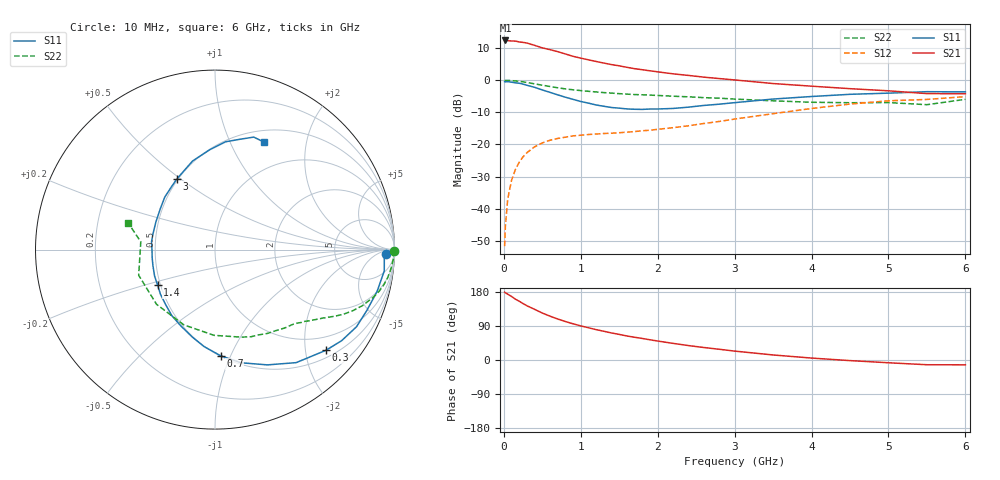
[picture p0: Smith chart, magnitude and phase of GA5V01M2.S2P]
! Infineon Technologies  Discrete & RF Semiconductors
! BF775
! Si NPN RF Bipolar Junction Transistor in SOT23
! VCE = 5 V  IC = 1.2 mA
! Common Emitter S-Parameters:  May  1996
# GHz  S  MA  R  50
!  f  S11  S21  S12  S22
! GHz  MAG  ANG  MAG  ANG  MAG  ANG  MAG  ANG
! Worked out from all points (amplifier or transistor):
!   36 points, 10 MHz to 6 GHz, reference 50 ohm
!   highest |S21| = 12.4 dB at 20 MHz (marker M1)
!   |S21| within 3 dB of that: start of sweep to 622.2 MHz
!   unconditionally stable (mu >= 1): 1.385 GHz to 3.704 GHz; 5.262 GHz to end of sweep
!   at 250 MHz: K = 0.21, MSG = 17.8 dB, |S12| = -23.8 dB
!   at 1.4 GHz: K = 1.01, MAG = 10.1 dB, |S12| = -16.5 dB
!   at 6 GHz: K = 1.00, MAG = 0.3 dB, |S12| = -5.1 dB
!   S11 on the Smith chart (normalised r, x): 10 MHz: 32, -17; 300 MHz: 0.66, -2.44; 700 MHz: 0.50, -0.92; 1.4 GHz: 0.48, -0.22; 3 GHz: 0.49, +0.48; 6 GHz: 0.64, +1.35
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0.01  0.9516 -1.5  4.094 179.0  0.0026 88.5  0.9999 -0.5
0.02  0.9444 -2.7  4.165 177.4  0.0053 92.0  0.9907 -1.2
0.05  0.9505 -7.2  4.133 173.8  0.014 85.1  0.9946 -3.1
0.1  0.9326 -14.5  4.084 167.7  0.0276 81.3  0.9867 -6.0
0.15  0.9113 -21.9  4.071 160.6  0.0406 76.4  0.975 -9.2
0.3  0.8349 -42.2  3.798 143.1  0.0744 65.2  0.9208 -16.8
0.4  0.7754 -54.3  3.493 133.7  0.0917 58.7  0.8779 -20.9
0.5  0.7058 -65.5  3.193 123.9  0.1055 53.5  0.8375 -24.1
0.6  0.6472 -77.0  2.996 115.6  0.1162 49.2  0.7986 -26.9
0.7  0.5921 -87.0  2.788 108.2  0.124 45.9  0.7631 -29.1
0.8  0.5438 -96.4  2.565 101.5  0.1297 43.1  0.7325 -31.0
0.9  0.5035 -104.5  2.358 95.5  0.1359 41.1  0.7094 -32.6
1.1  0.4398 -123.1  2.079 85.1  0.1427 38.7  0.6726 -35.7
1.4  0.3757 -148.5  1.752 71.3  0.1495 37.8  0.6301 -40.1
1.7  0.353 -172.6  1.514 60.0  0.1586 39.6  0.598 -44.5
2.2  0.3635 155.0  1.258 43.9  0.1823 43.5  0.5636 -53.4
3  0.4474 118.4  1.011 23.5  0.2482 46.3  0.5089 -73.4
3.5  0.5093 104.2  0.888 13.3  0.3014 44.0  0.4778 -90.6
4.5  0.6035 84.4  0.739 -1.6  0.4251 32.9  0.4461 -136.9
5  0.6292 77.5  0.684 -7.3  0.4783 24.8  0.4486 -161.4
5.5  0.6629 71.0  0.619 -12.5  0.5024 15.6  0.4158 174.0
6  0.6584 65.4  0.616 -12.7  0.5552 10.8  0.5042 163.1
